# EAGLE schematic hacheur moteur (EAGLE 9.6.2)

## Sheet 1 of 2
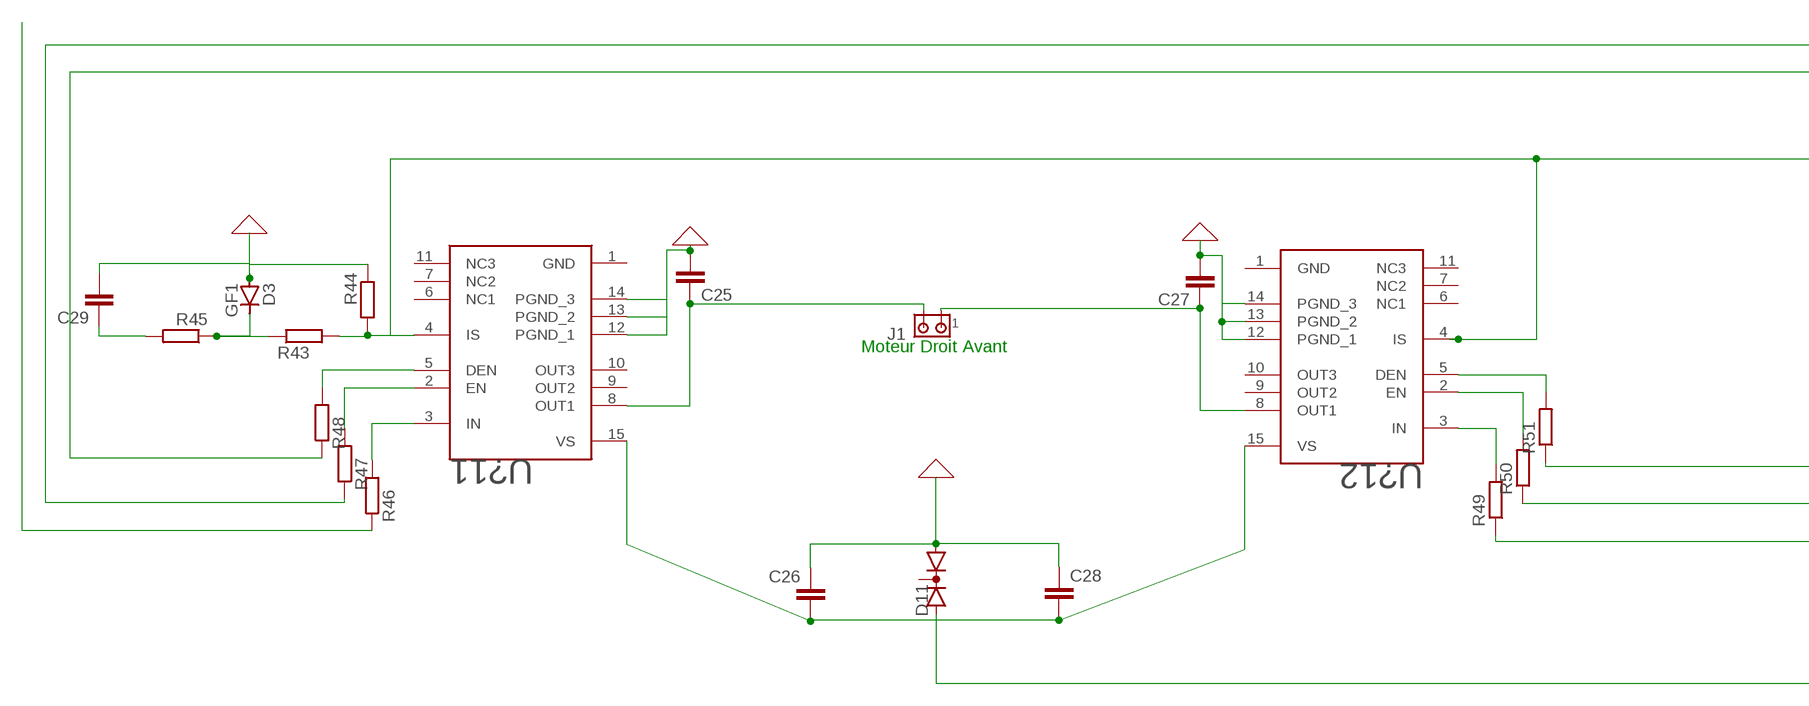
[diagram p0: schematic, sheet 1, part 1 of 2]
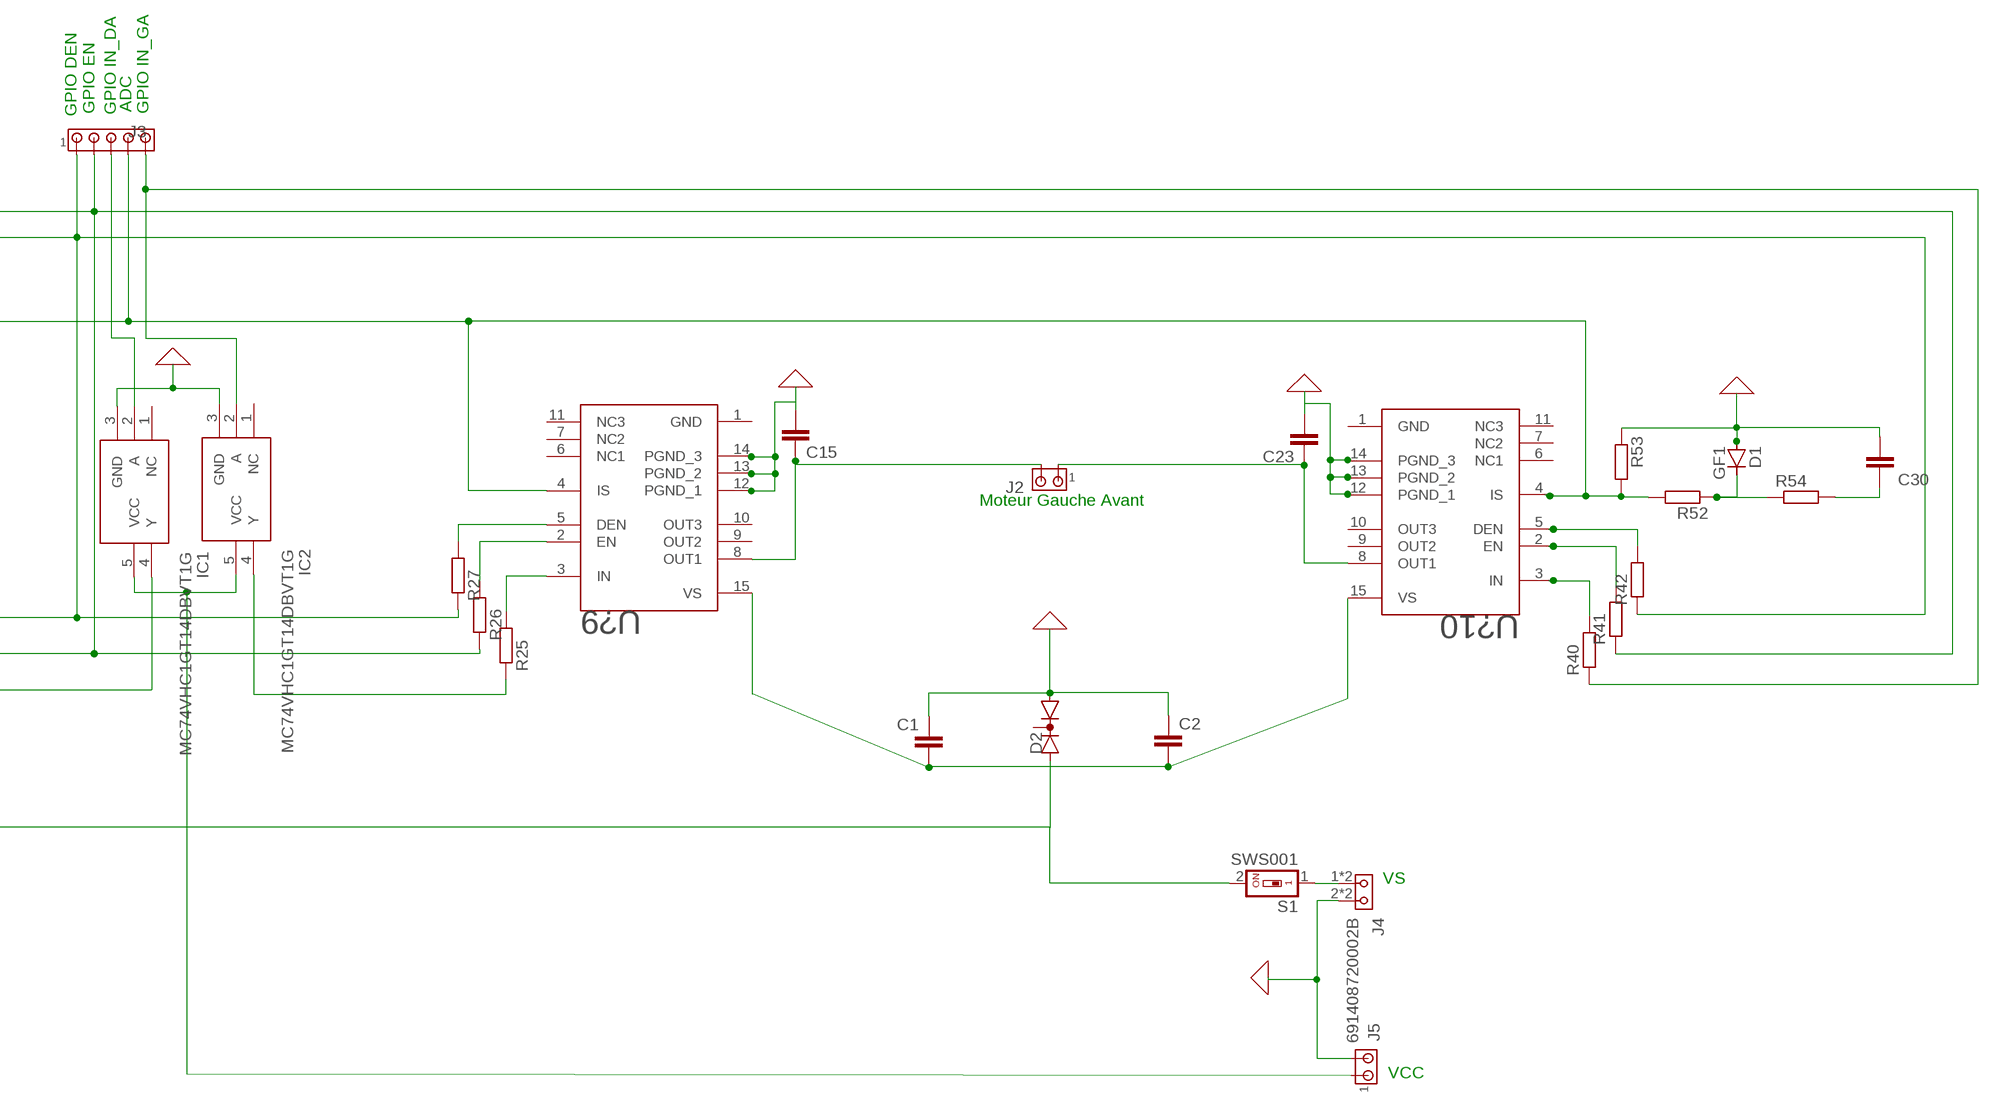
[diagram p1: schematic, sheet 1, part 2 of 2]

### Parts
C1  C-EUC1206K  [C1206K]
C2  C-EUC1206K  [C1206K]
C15  C-EUC1206K  [C1206K]
C23  C-EUC1206K  [C1206K]
C25  C-EUC1206K  [C1206K]
C26  C-EUC1206K  [C1206K]
C27  C-EUC1206K  [C1206K]
C28  C-EUC1206K  [C1206K]
C29  C-EUC1206K  [C1206K]
C30  C-EUC1206K  [C1206K]
D1  GF1  [SMA-DO214AC]
D2  DIODE_AC-CA_  [SOT23C]
D3  GF1  [SMA-DO214AC]
D11  DIODE_AC-CA_  [SOT23C]
IC1  MC74VHC1GT14DBVT1G  [SOT95P275X110-5N]
IC2  MC74VHC1GT14DBVT1G  [SOT95P275X110-5N]
J1  MTA02-156  [1X2MTA]
J2  MTA02-156  [1X2MTA]
J3  MTA05-156  [1X5MTA]
J4  691408720002B  [691408720002B]
J5  MTA02-100  [10X02MTA]
R25  R-EU_R1206W  [R1206W]
R26  R-EU_R1206W  [R1206W]
R27  R-EU_R1206W  [R1206W]
R40  R-EU_R1206W  [R1206W]
R41  R-EU_R1206W  [R1206W]
R42  R-EU_R1206W  [R1206W]
R43  R-EU_R1206W  [R1206W]
R44  R-EU_R1206W  [R1206W]
R45  R-EU_R1206W  [R1206W]
R46  R-EU_R1206W  [R1206W]
R47  R-EU_R1206W  [R1206W]
R48  R-EU_R1206W  [R1206W]
R49  R-EU_R1206W  [R1206W]
R50  R-EU_R1206W  [R1206W]
R51  R-EU_R1206W  [R1206W]
R52  R-EU_R1206W  [R1206W]
R53  R-EU_R1206W  [R1206W]
R54  R-EU_R1206W  [R1206W]
S1  SWS001  [SMS-001]
U?9  BTN7030-1EPA  [SOP65P600X115-15N-V]
U?10  BTN7030-1EPA  [SOP65P600X115-15N-V]
U?11  BTN7030-1EPA  [SOP65P600X115-15N-V]
U?12  BTN7030-1EPA  [SOP65P600X115-15N-V]

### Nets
0: C1.1 C2.1 C15.2 C23.2 C25.2 C26.1 C27.2 C28.1 C29.2 C30.2 D1.A D2.1(A1) D3.A D11.1(A1) IC1.3(GND) IC2.3(GND) J4.2 J4.A2 J5.2 R44.1 R53.1 U?11.12(PGND_1) U?11.13(PGND_2) U?11.14(PGND_3) U?12.12(PGND_1) U?12.13(PGND_2) U?12.14(PGND_3) ; supply symbol labelled GND
N$1: R48.2 U?11.5(DEN)
N$2: R47.2 U?11.2(EN)
N$3: D3.K(C) R43.1 R45.1
N$4: IC1.4(Y) R49.1
N$5: J4.1 J4.A1 S1.1
N$6: C1.2
N$7: C2.2
N$8: U?9.15(VS)
N$9: IC1.2(A) J3.3
N$10: R46.1
N$11: IC2.4(Y) R25.1
N$13: IC1.5(VCC) IC2.5(VCC) J5.1
N$92: C15.1 J2.2 U?9.8(OUT1)
N$93: C23.1 J2.1 U?10.8(OUT1)
N$96: R25.2 U?9.3(IN)
N$97: R26.2 U?9.2(EN)
N$98: R27.2 U?9.5(DEN)
N$99: R40.2 U?10.3(IN)
N$100: R41.2 U?10.2(EN)
N$101: R42.2 U?10.5(DEN)
N$102: C26.2 U?11.15(VS)
N$103: C25.1 J1.2 U?11.8(OUT1)
N$104: C27.1 J1.1 U?12.8(OUT1)
N$105: C28.2 U?12.15(VS)
N$107: R43.2 R44.2 U?11.4(IS)
N$109: C29.1 R45.2
N$110: U?12.4(IS)
N$112: R46.2 U?11.3(IN)
N$113: R51.2 U?12.5(DEN)
N$114: R50.2 U?12.2(EN)
N$115: R49.2 U?12.3(IN)
N$118: IC2.2(A) J3.5 R40.1
N$119: J3.2 R26.1 R41.1 R47.1 R50.1
N$120: J3.1 R27.1 R42.1 R48.1 R51.1
N$121: U?10.4(IS)
N$122: R52.2 R53.2
N$123: D1.K(C) R52.1 R54.1
N$124: C30.1 R54.2
N$126: J3.4
PROTECTION1: D11.2(A2) S1.2
PROTECTION2: D2.2(A2)
Unconnected: D2.3(K) D11.3(K) IC1.1(NC) IC2.1(NC) U?9.4(IS) U?9.6(NC1) U?9.7(NC2) U?9.9(OUT2) U?9.10(OUT3) U?9.11(NC3) U?10.6(NC1) U?10.7(NC2) U?10.9(OUT2) U?10.10(OUT3) U?10.11(NC3) U?11.6(NC1) U?11.7(NC2) U?11.9(OUT2) U?11.10(OUT3) U?11.11(NC3) U?12.6(NC1) U?12.7(NC2) U?12.9(OUT2) U?12.10(OUT3) U?12.11(NC3)

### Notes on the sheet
- GPIO DEN | GPIO EN | GPIO IN_DA | ADC | GPIO IN_GA
- Moteur Droit Avant | Moteur Gauche Avant
- VS
- VCC

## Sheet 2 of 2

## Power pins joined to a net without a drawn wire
GND: U?9.1(GND) U?10.1(GND) U?11.1(GND) U?12.1(GND)
PGND_1: U?9.12(PGND_1) U?10.12(PGND_1)
PGND_2: U?9.13(PGND_2) U?10.13(PGND_2)
PGND_3: U?9.14(PGND_3) U?10.14(PGND_3)
VS: U?10.15(VS)

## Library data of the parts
C1 C2 C15 C23 C25-C30 = rcl:C-EU: CAPACITOR, European symbol; SPICEPREFIX: C
D1 D3 = diode:GF1: DIODE
D2 D11 = semicon-smd-ipc:DIODE_AC-CA_: DUAL DIODE
IC1 IC2 = MC74VHC1GT14DBVT1G:MC74VHC1GT14DBVT1G: ON SEMICONDUCTOR - MC74VHC1GT14DBVT1G - Logic IC, Inverter, Single, 1 Inputs, 5 Pins, SC-74A, 74VHC1GT14 Source: Datasheet; ARROW_PART_NUMBER: MC74VHC1GT14DBVT1G; ARROW_PRICE-STOCK: https://www.arrow.com/en/products/mc74vhc1gt14dbvt1g/on-semiconductor?region=nac; DESCRIPTION: ON SEMICONDUCTOR - MC74VHC1GT14DBVT1G - Logic IC, Inverter, Single, 1 Inputs, 5 Pins, SC-74A, 74VHC1GT14; HEIGHT: 1.1mm; MANUFACTURER_NAME: onsemi; MANUFACTURER_PART_NUMBER: MC74VHC1GT14DBVT1G; MOUSER_PART_NUMBER: 863-MC74VHC1GT14DBVG; MOUSER_PRICE-STOCK: https://www.mouser.co.uk/ProductDetail/onsemi/MC74VHC1GT14DBVT1G?qs=vLWxofP3U2y98PQgYBav%252Bw%3D%3D
J1 J2 = con-amp:MTA02-156: AMP connector
J3 = con-amp:MTA05-156: AMP connector
J4 = Wurth_Connectors_WR-TBL Spring Clamp:691408720002B: WR-TBL Series 4087B - Screwless Push In 5.0mm pitch - 45° cable entry - THT; DATASHEET-URL: https://www.we-online.com/catalog/datasheet/691408720002B.pdf; IR-UL: 15A; MOUNT: THT; PART-NUMBER: 691408720002B; PINS: 2; PITCH: 5mm; TYPE: 45° Cable Entry; WIRE: 28 to 12 (AWG) 0.2 to 2.5 (mm²); WORKING-VOLTAGE-UL: 300V (AC)
J5 = con-amp:MTA02-100: AMP connector
R25-R27 R40-R54 = rcl:R-EU_: RESISTOR, European symbol; SPICEPREFIX: R
S1 = smd-special:SWS001: SMD Dip Switch 1 pol.
U?9-U?12 = BTN7030-1EPA:BTN7030-1EPA: BTN7030-1EPA SOP65P600X115-15N-V NovalithIC Lite Integrated Half Bridge

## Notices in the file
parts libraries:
Wurth_Connectors_WR-TBL Spring Clamp: Copyright: Würth Elektronik
